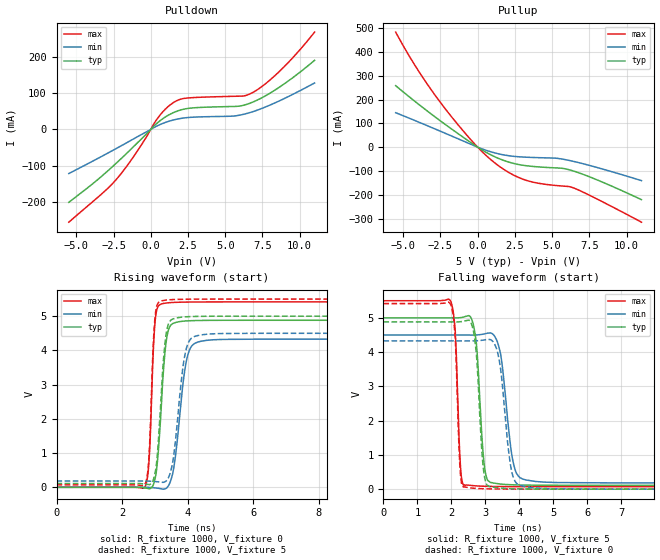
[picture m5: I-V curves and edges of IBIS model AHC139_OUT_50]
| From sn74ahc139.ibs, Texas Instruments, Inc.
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[Model]   AHC139_OUT_50
Model_type  Output
Vref =   0
Rref =   1000
Cref =   50p
Vmeas =   2.5
| variable   typ   min   max
C_comp   2.28pF   1.71pF   3.25pF
| C_pullup   2.53pF   1.80pF   3.25pF
| C_pulldown   2.03pF   1.71pF   2.44pF
[Temperature Range]   40   100   -40
| Ambient temperature   25   85   -40
[Voltage range]   5   4.5   5.5
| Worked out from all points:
|   slope of the pulldown table from 0 to 0.75 V, typ, clamps not added: 26.9 ohm
|   slope of the pullup table from 0 to 0.75 V, typ, clamps not added: 26.8 ohm
|   rising waveform, R_fixture 1000, V_fixture 0: 20-80 % time 206ps typ, 299ps min, 130ps max; typ from 0 V to 4.88 V
|   falling waveform, R_fixture 1000, V_fixture 5: 20-80 % time 176ps typ, 278ps min, 117ps max; typ from 5 V to 0.112 V
|   rising waveform, R_fixture 1000, V_fixture 5: 20-80 % time 203ps typ, 285ps min, 130ps max; typ from 0.112 V to 5 V
|   falling waveform, R_fixture 1000, V_fixture 0: 20-80 % time 168ps typ, 262ps min, 113ps max; typ from 4.88 V to 0 V
[Pulldown]
| AHC139_OUT_50
|   Voltage   I(typ)   I(min)   I(max)
-5.5V     -201.8mA   -122.2mA   -256.8mA
-2.325V   -93.87mA   -53.16mA   -139.1mA
-1.065V   -44.23mA   -24.29mA   -70.11mA
475mV     18.91mA    10.47mA    31.51mA
1.315V    42.25mA    23.7mA     68.09mA
2.285V    56.53mA    31.87mA    85.91mA
5.56V     63.43mA    36.87mA    91.53mA
6.265V    67.11mA    42.03mA    92.71mA
6.75V     73.82mA    47.63mA    99.98mA
7.61V     90.82mA    60.43mA    123.3mA
8.665V    117.6mA    79.47mA    161.5mA
11V       191.2mA    128.4mA    269.2mA
[Pullup]
| AHC139_OUT_50
|   Voltage   I(typ)   I(min)   I(max)
-5.5V     258.1mA    144.6mA    483.2mA
-4.005V   182.1mA    106.4mA    323.6mA
-2.335V   102.7mA    62.37mA    174.2mA
-295mV    12.38mA    7.743mA    19.77mA
475mV     -18.46mA   -11.39mA   -29.55mA
1.225V    -42.56mA   -25.5mA    -69.79mA
2.265V    -66.01mA   -37.62mA   -112.6mA
3.31V     -78.54mA   -42.51mA   -140.4mA
5.25V     -87.39mA   -46.53mA   -161.2mA
6.28V     -97.54mA   -57.77mA   -167.9mA
8.105V    -139.9mA   -87.12mA   -220.8mA
11V       -220.7mA   -140.8mA   -315.4mA
[Ramp]
| AHC139_OUT_50
| variable   typ   min   max
dV/dt_r   2.96/2.16E-10   2.63/3.13E-10   3.27/1.35E-10
dV/dt_f   2.97/1.85E-10   2.63/2.94E-10   3.29/1.24E-10
R_load = 1000
[Rising Waveform]
| AHC139_OUT_50
R_fixture =   1000
C_fixture =   0
L_fixture =   0
V_fixture =   0
V_fixture_min = 0
V_fixture_max = 0
|   Time   V(typ)   V(min)   V(max)
0s        1.434nV    2.383nV    883pV
2.695ns   -18.93mV   1.402mV    2.643mV
2.825ns   -42.08mV   -2.827mV   813.9mV
2.955ns   77.15mV    -12.27mV   4.02V
3.02ns    309.3mV    -18.32mV   4.957V
3.335ns   4.172V     -35.48mV   5.383V
3.58ns    4.797V     584.9mV    5.402V
4.005ns   4.864V     3.863V     5.412V
4.575ns   4.877V     4.293V     5.416V
40ns      4.88V      4.329V     5.417V
[Falling Waveform]
| AHC139_OUT_50
R_fixture =   1000
C_fixture =   0
L_fixture =   0
V_fixture =   5
V_fixture_min = 4.5
V_fixture_max = 5.5
|   Time   V(typ)   V(min)   V(max)
0s        5V         4.5V       5.5V
1.98ns    4.999V     4.5V       5.487V
2.11ns    4.999V     4.5V       4.657V
2.36ns    5.025V     4.499V     115.9mV
2.71ns    4.434V     4.5V       97.06mV
3ns       479.8mV    4.538V     84.17mV
3.39ns    156.7mV    4.176V     77.31mV
3.855ns   126.1mV    627.3mV    74.34mV
4.46ns    116.2mV    225.6mV    73.05mV
40ns      112.1mV    183.3mV    72.37mV
[Rising Waveform]
| AHC139_OUT_50
R_fixture =   1000
C_fixture =   0
L_fixture =   0
V_fixture =   5
V_fixture_min = 4.5
V_fixture_max = 5.5
|   Time   V(typ)   V(min)   V(max)
0s        112.1mV    183.3mV    72.37mV
2.695ns   94.56mV    184.1mV    81.24mV
2.815ns   79.22mV    180.4mV    810.6mV
2.945ns   189.9mV    172.3mV    4.021V
3.015ns   459.1mV    167.3mV    5.051V
3.325ns   4.335V     171.3mV    5.468V
3.55ns    4.918V     757mV      5.485V
3.965ns   4.982V     4.067V     5.496V
4.5ns     4.996V     4.464V     5.499V
40ns      5V         4.5V       5.5V
[Falling Waveform]
| AHC139_OUT_50
R_fixture =   1000
C_fixture =   0
L_fixture =   0
V_fixture =   0
V_fixture_min = 0
V_fixture_max = 0
|   Time   V(typ)   V(min)   V(max)
0s        4.88V      4.329V     5.417V
1.98ns    4.88V      4.329V     5.389V
2.355ns   4.902V     4.328V     62.14mV
2.66ns    4.544V     4.328V     27.19mV
2.94ns    596.1mV    4.351V     13.15mV
3.135ns   69.91mV    4.369V     8.389mV
3.415ns   35.91mV    3.708V     4.638mV
3.8ns     14.16mV    406.7mV    2.209mV
4.36ns    4.598mV    45.83mV    826.9uV
40ns      -4.14nV    -6.059nV   -513.7pV
